(* Logix 5000 AddOnInstructionDefinition export Banner_RCD; software revision 33.00 *)

ADD_ON_INSTRUCTION Banner_RCD   (* revision 1.2 *)
// AOI that activates a Reset or Cancel Delay operation to a Banner XS26 or SC26.
// Revision note:
// Add Bit.0 check on rung 3 to handle a sequence issue that was encountered. Ensures that Rung 0 has run before allowing the code to be turned off.
VAR_INPUT
   RCD_Code : INT; {required}
END_VAR
VAR_IN_OUT
   RCD_Act_Code : INT; {required}
   RCD_Act_FB : INT; {required}
   RCD_Bit : BOOL; {required}
   Control_Bit : BOOL; {required}
END_VAR
VAR_OUTPUT
   Error : DINT;
   Act_Sent : DINT;
   Act_Recevied : DINT;
END_VAR
VAR
   Bit : DINT; {access None}
   Timer : TIMER := (PRE := 3000); {access None}
END_VAR

ROUTINE Logic   (* ladder *)
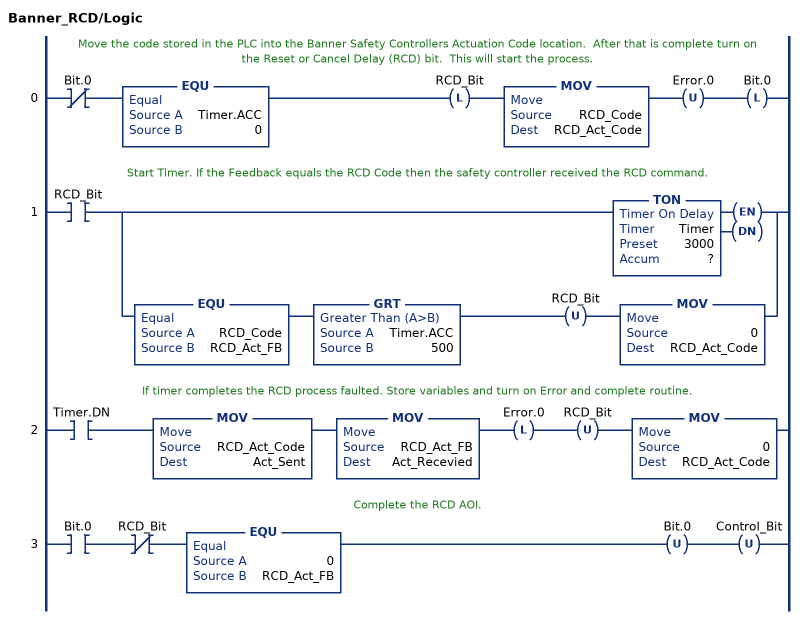
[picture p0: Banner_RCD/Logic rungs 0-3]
   // Move the code stored in the PLC into the Banner Safety Controllers Actuation Code location.  After that is complete turn on the Reset or Cancel Delay (RCD) bit.  This will start the process.
   0: XIO(Bit.0)EQU(Timer.ACC,0)OTL(RCD_Bit)MOV(RCD_Code,RCD_Act_Code)OTU(Error.0)OTL(Bit.0);
   // Start Timer. If the Feedback equals the RCD Code then the safety controller received the RCD command.
   1: XIC(RCD_Bit)[TON(Timer,?,?) ,EQU(RCD_Code,RCD_Act_FB) GRT(Timer.ACC,500) OTU(RCD_Bit) MOV(0,RCD_Act_Code) ];
   // If timer completes the RCD process faulted. Store variables and turn on Error and complete routine.
   2: XIC(Timer.DN)MOV(RCD_Act_Code,Act_Sent)MOV(RCD_Act_FB,Act_Recevied)OTL(Error.0)OTU(RCD_Bit)MOV(0,RCD_Act_Code);
   // Complete the RCD AOI.
   3: XIC(Bit.0)XIO(RCD_Bit)EQU(0,RCD_Act_FB)OTU(Bit.0)OTU(Control_Bit);
END_ROUTINE
END_ADD_ON_INSTRUCTION
